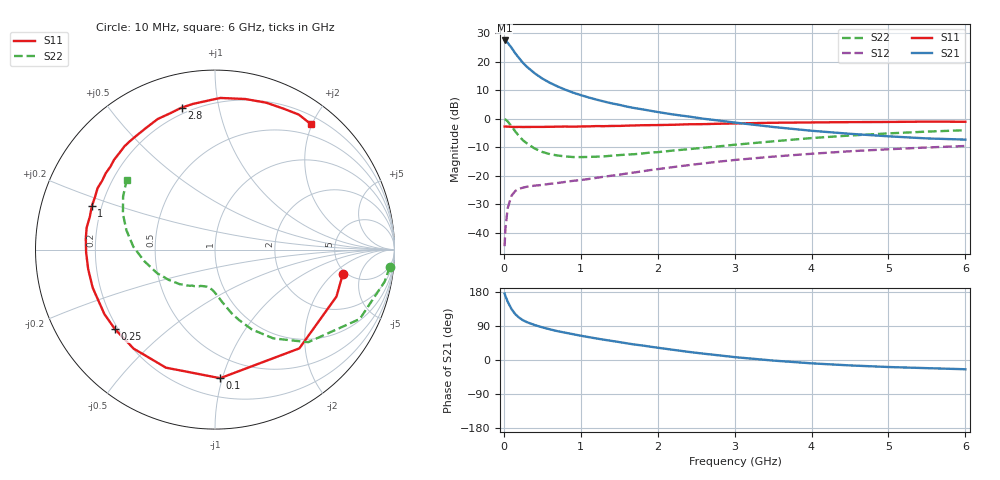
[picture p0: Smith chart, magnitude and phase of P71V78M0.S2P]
! SIEMENS Small Signal Semiconductors
! BFP196
! Si NPN RF Bipolar Junction Transistor in SOT143
! VCE = 1.75 V  IC = 8 mA
! Common Emitter S-Parameters:  May  1996
# GHz  S  MA  R  50
!  f  S11  S21  S12  S22
! GHz  MAG  ANG  MAG  ANG  MAG  ANG  MAG  ANG
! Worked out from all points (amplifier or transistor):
!   36 points, 10 MHz to 6 GHz, reference 50 ohm
!   highest |S21| = 27.4 dB at 10 MHz (marker M1)
!   |S21| within 3 dB of that: start of sweep to 111.4 MHz
!   unconditionally stable (mu >= 1): 930.9 MHz to 3.305 GHz
!   at 250 MHz: K = 0.35, MSG = 21.9 dB, |S12| = -24.2 dB
!   at 1.4 GHz: K = 1.16, MAG = 10.3 dB, |S12| = -20.0 dB
!   at 6 GHz: K = 0.99, MSG = 1.1 dB, |S12| = -9.6 dB
!   S11 on the Smith chart (normalised r, x): 10 MHz: 4.66, -2.70; 100 MHz: 0.33, -0.98; 250 MHz: 0.19, -0.34; 1 GHz: 0.16, +0.17; 2.8 GHz: 0.17, +0.78; 6 GHz: 0.32, +1.99
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0.01  0.7251 -10.9  23.42 175.4  0.0058 86.9  0.9786 -5.6
0.02  0.7256 -21.1  22.81 168.8  0.0117 79.7  0.962 -10.7
0.05  0.7237 -49.5  21.32 154.0  0.027 67.0  0.8945 -25.6
0.1  0.717 -87.7  17.48 134.4  0.0446 50.5  0.7319 -44.8
0.15  0.7124 -112.6  13.87 120.7  0.0539 41.1  0.5919 -56.7
0.2  0.714 -129.4  11.41 111.6  0.0589 35.4  0.49 -65.2
0.25  0.7122 -141.4  9.459 104.8  0.0616 31.6  0.4152 -71.1
0.3  0.7134 -149.7  8.072 99.9  0.0639 30.4  0.3673 -75.3
0.4  0.7138 -162.7  6.243 92.3  0.0668 28.7  0.2992 -81.7
0.5  0.715 -171.3  5.033 86.2  0.0687 28.7  0.2598 -86.7
0.6  0.7182 -178.7  4.231 80.9  0.0719 29.6  0.2379 -90.5
0.7  0.7223 175.2  3.654 76.0  0.0743 30.7  0.2249 -93.8
0.8  0.7256 170.3  3.205 72.0  0.0777 31.7  0.2174 -97.0
1  0.7276 160.6  2.581 64.1  0.0836 34.8  0.2114 -102.9
1.1  0.73 156.4  2.35 60.5  0.0872 36.2  0.2127 -105.9
1.6  0.7529 138.3  1.62 44.0  0.109 40.2  0.2339 -119.5
2.2  0.7788 119.7  1.181 26.9  0.1411 40.3  0.2749 -135.4
2.8  0.8127 103.2  0.922 12.2  0.1762 37.0  0.3263 -152.7
3.5  0.8454 88.0  0.713 -1.5  0.2154 30.2  0.3992 -170.7
4.5  0.8668 70.8  0.541 -14.3  0.2675 19.2  0.5051 167.7
5.5  0.8852 58.2  0.449 -21.5  0.3116 7.7  0.5912 150.0
6  0.8798 52.4  0.428 -24.4  0.331 1.4  0.6255 142.0
